PROGRAM MAIN
VAR
	Axis1	: AXIS_REF;
	
	fbPower	: MC_Power;
	
	fbHome	: FB_DiverBasedHoming;
END_VAR


fbPower.Enable			;
fbPower.Enable_Positive	:= TRUE;  
fbPower.Enable_Negative	:= TRUE; 
fbPower( Axis := Axis1 );

fbHome.stParameter.Acceleration := 5000;
fbHome.stParameter.HomeMethod	:= 1;
fbHome.stParameter.HomeOffset	:= -10;
fbHome.stParameter.VelocityForSwitch:= 10;
fbHome.stParameter.VelocityForIndex := 1;
fbHome( AxisRef := Axis1 );

END_PROGRAM
